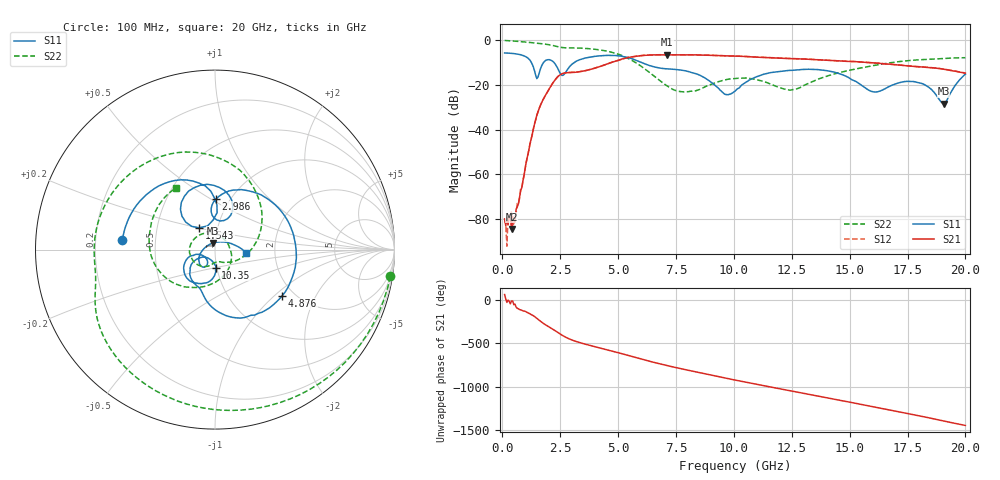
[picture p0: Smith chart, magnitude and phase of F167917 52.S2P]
!  2-Port S-parameters saved by WinCal
! VAR MeasName=S-Parameters (CALIBRATED_DATA) read from VNA (N5242A)
! VAR MeasDate=2016-11-22 9:02:28
! VAR NAME=F167917 52
! VAR FILENAME=F167917 52.S2P
! VAR DATE=2016-11-22 9:02:28
! VAR PHYS_PORTS=1,2
# Hz S DB R 50
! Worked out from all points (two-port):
!   401 points, 100 MHz to 20 GHz, reference 50 ohm
!   highest |S21| = -6.50 dB at 7.115 GHz (marker M1); lowest = -84.5 dB at 398.5 MHz (marker M2)
!   |S21| within 3 dB of the highest: 4.85 GHz to 14.96 GHz (10.11 GHz wide, 102 % of centre); 15.05033 GHz to 15.09133 GHz (41 MHz wide, 0.272 % of centre)
!   lowest |S11| = -28.4 dB at 19.05 GHz (marker M3), VSWR 1.08, Z = 48.8 + j3.58 ohm
!   |S11| at or under -10 dB: 1.256 GHz to 1.781 GHz (524.2 MHz wide, 34.5 % of centre); 2.234 GHz to 3.109 GHz (874.6 MHz wide, 32.7 % of centre); 6.019 GHz to end of sweep
!   |S22| runs from -23.1 to -0.1 dB; largest |S21 - S12| = 0.0038
!   S11 on the Smith chart (normalised r, x): 100 MHz: 0.32, +0.05; 1.543 GHz: 0.82, +0.20; 2.986 GHz: 0.86, +0.53; 4.876 GHz: 1.73, -1.13; 10.35 GHz: 0.99, -0.20; 20 GHz: 1.42, -0.05
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1e8  -5.71 174.2  -80.05 62.5  -79.87 64.3  -0.10 -8.7
3.985e8  -5.88 156.5  -84.51 -11.0  -76.64 -24.0  -0.29 -32.9
6.4725e8  -6.21 141.1  -74.59 -95.9  -73.12 -98.8  -0.48 -52.2
1.54275e9  -16.48 126.0  -32.06 137.4  -32.05 137.8  -1.38 -112.9
1.94075e9  -8.78 108.6  -23.28 61.8  -23.27 61.9  -1.89 -136.0
2.5875e9  -15.80 79.8  -15.01 -46.5  -14.99 -46.4  -3.28 -165.9
2.9855e9  -10.96 88.7  -14.42 -98.6  -14.41 -98.6  -3.44 179.5
3.43325e9  -8.44 59.5  -13.95 -138.0  -13.95 -138.0  -3.57 160.2
4.876e9  -6.85 -34.5  -9.42 121.6  -9.42 121.8  -5.84 87.6
5.72175e9  -8.78 -82.7  -7.27 59.3  -7.24 59.4  -9.79 36.1
6.7665e9  -12.40 -109.0  -6.52 -13.1  -6.50 -13.1  -17.78 -29.3
7.11475e9  -12.81 -113.7  -6.50 -35.3  -6.49 -35.2  -20.44 -48.7
8.3585e9  -15.01 -141.2  -6.58 -108.8  -6.54 -108.7  -22.66 -95.4
1.005e10  -22.82 -96.8  -7.08 158.0  -7.09 158.1  -17.20 -159.1
1.03485e10  -20.00 -87.5  -7.21 141.8  -7.17 141.9  -16.90 -172.5
1.1642e10  -14.43 -104.2  -7.88 74.8  -7.83 74.8  -19.82 113.7
1.338325e10  -13.05 -133.7  -8.63 -14.3  -8.59 -14.4  -18.59 -43.5
1.497525e10  -16.85 -165.1  -9.51 -95.2  -9.49 -95.6  -13.50 -104.8
1.67165e10  -20.73 -117.6  -10.69 173.2  -10.73 173.3  -10.15 -147.7
1.805975e10  -19.20 -144.4  -11.93 103.0  -11.88 103.1  -8.73 177.2
1.905475e10  -28.36 106.5  -12.96 47.3  -12.94 47.1  -8.17 151.1
2e10  -15.20 -5.6  -14.75 -4.9  -14.67 -4.6  -7.84 122.3
